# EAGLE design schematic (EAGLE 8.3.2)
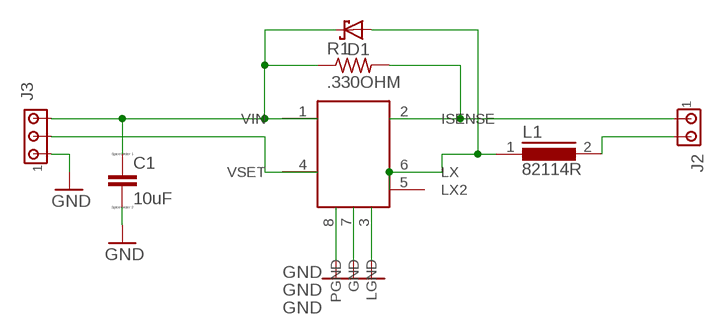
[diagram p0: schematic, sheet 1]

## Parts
C1  10uF  CC1206  [C1206]
D1  SCHOTTKY-DIODESMC  [SMC]
J2  MTA02-156  [1X2MTA]
J3  MTA03-156  [1X3MTA]
L1  82114R  [82114R]
R1  .330OHM  R-US_0207/15  [0207/15]
U$1  PAM2863  [SOP8]

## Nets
GND: C1.2 J3.1 U$1.3(LGND) U$1.7(GND) U$1.8(PGND)
LED+: J2.1 R1.2 U$1.2(ISENSE)
LED-: J2.2 L1.2
N$5: D1.A L1.1 U$1.5(LX2) U$1.6(LX)
VIN: C1.1 D1.C J3.3 R1.1 U$1.1(VIN)
VSET: J3.2 U$1.4(VSET)

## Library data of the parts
C1 = eagle-ltspice:C: CAPACITOR, European symbol; SPICEMODEL: NONE; SPICEPREFIX: C
D1 = diode:SCHOTTKY-DIODE: Schottky Diode
J2 = con-amp:MTA02-156: AMP connector
J3 = con-amp:MTA03-156: AMP connector
L1 = inductors:82114R: INDUCTOR
R1 = rcl:R-US_: RESISTOR, American symbol
U$1 = raccolta:PAM2863: The PAM2863 is a continuous mode inductive step-down converter, designed for driving single or multiple series connected LEDs efficiently from a voltage source higher than the LED voltage. The device operates from an input supply between 4.5V and 40V and provides an externally adjustable output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

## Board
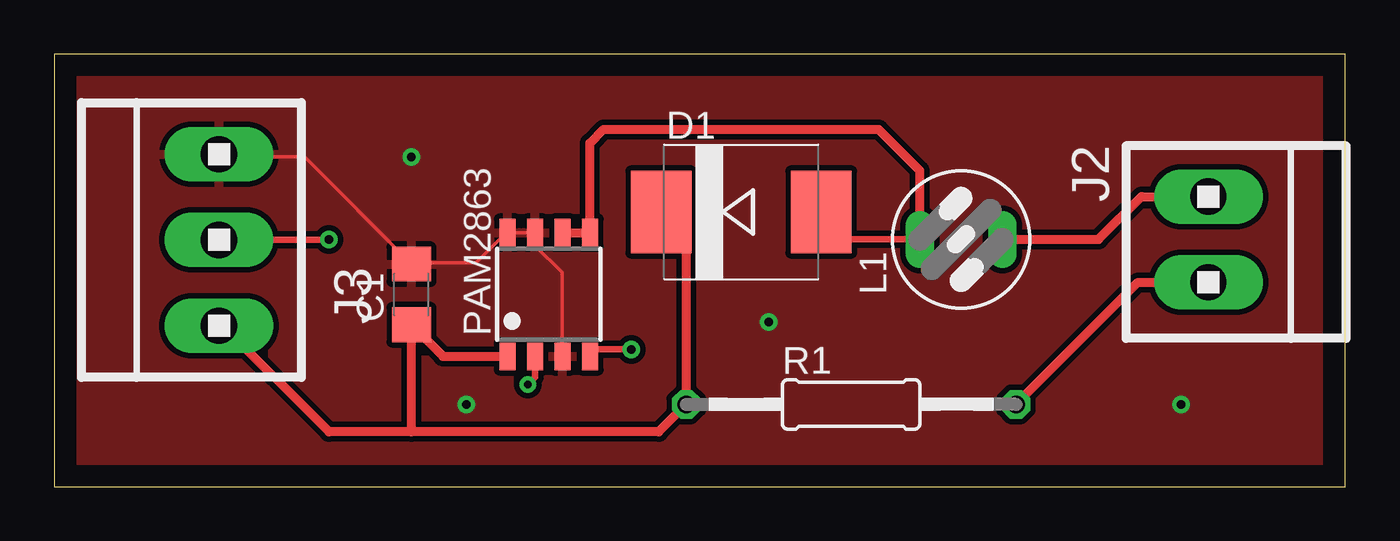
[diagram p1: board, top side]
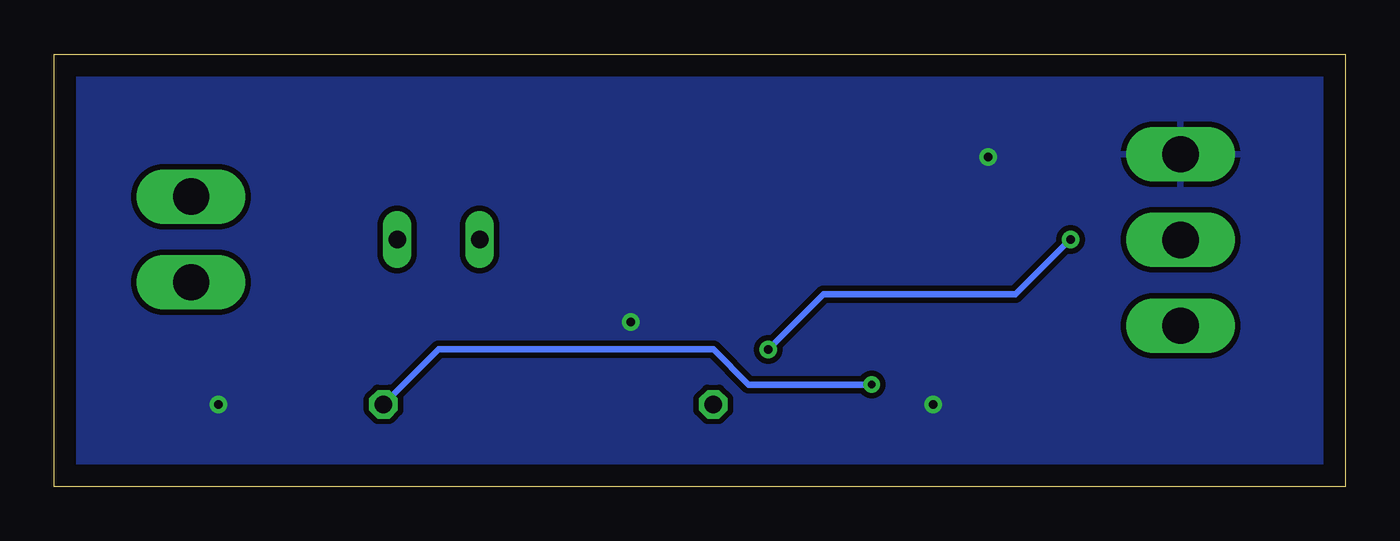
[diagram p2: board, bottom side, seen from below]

Size 59.67 x 19.99 mm. Coordinates in mm from the lower left corner, seen from the top.
Outline: 0,0 59.67,0 59.67,19.99 0,19.99 0,0
Copper layers (1*16): Top 0.035mm / dielectric 1.5mm / Bottom 0.035mm
Design rules "default": minimum track width 6mil, minimum drill 0.35mm, track to track 6mil, track to pad 6mil, pad to pad 6mil, via to via 6mil, smd to smd 6mil, copper to edge 40mil, drill to drill 6mil, minimum pad ring 10mil, minimum via ring 8mil, stop-mask expansion 4mil, vias tented up to drill 0mil, thermal gap 10mil

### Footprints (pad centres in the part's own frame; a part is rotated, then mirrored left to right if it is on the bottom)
C1206 = smd 1.6 x 1.8: 1 -1.4,0; 2 1.4,0
SMC = smd 2.8 x 3.8: A 3.7,0; C -3.7,0
1X2MTA = drill 1.676 long: 1 1.981,0; 2 -1.981,0
1X3MTA = drill 1.676 long: 1 3.937,0; 2 -0.025,0; 3 -3.988,0
82114R = drill 0.813 long: 1 0,1.905; 2 0,-1.905
0207/15 = drill 0.813 octagon: 1 -7.62,0; 2 7.62,0
SOP8 = smd 0.76 x 1.27: 1 -1.905,-2.86; 2 -0.635,-2.86; 3 0.635,-2.86; 4 1.905,-2.86; 5 1.905,2.86; 6 0.635,2.86; 7 -0.635,2.86; 8 -1.905,2.86

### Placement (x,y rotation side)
C1  16.51,8.89 90 top
D1  31.75,12.7 0 top
J2  53.34,11.43 270 top
J3  7.62,11.43 90 top
L1  41.91,11.43 90 top
R1  36.83,3.81 0 top
U$1  22.86,8.89 0 top

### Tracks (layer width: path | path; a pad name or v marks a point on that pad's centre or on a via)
GND  (via drill 0.4)
  Top 0.152: U$1.3 23.47,6.1 23.47,9.91 22.25,11.12 22.25,11.73 U$1.7 22.1,11.73 21.03,11.73 U$1.8 20.88,11.73 19.51,10.36 16.61,10.36 C1.2 16.46,10.36 11.58,15.24 7.62,15.24 J3.1
  other vias: 16.51,15.24 33.02,7.62 19.05,3.81 52.07,3.81
  pour Top (isolate 0.254): 0,20.32 59.69,20.32 59.69,0 0,0
  pour Bottom (isolate 0.254): 0,0 0,20.32 59.69,20.32 59.69,0
LED+  (via drill 0.35)
  Top 0.305: v21.89,4.72 22.23,5.05 U$1.2
  Top 0.406: R1.2 50.09,9.45 J2.1
  Bottom 0.305: v21.89,4.72 27.58,4.72 29.21,6.35 41.91,6.35 R1.2
LED-
  Top 0.406: L1.2 48.26,11.43 50.24,13.41 J2.2
N$5
  Top 0.152: U$1.6 23.62,11.73 | 24.69,11.73 U$1.5
  Top 0.305: D1.A 36.72,11.43 L1.1
  Top 0.406: U$1.5 24.77,15.88 25.4,16.51 38.1,16.51 40.01,14.61 L1.1 | 23.62,11.73 24.69,11.73
VIN
  Top 0.406: D1.C 29.21,11.54 R1.1 27.94,2.54 16.51,2.54 | 16.51,2.54 12.7,2.54 7.8,7.44 J3.3 | 16.51,2.54 C1.1 17.97,6.03 U$1.1
VSET  (via drill 0.4)
  Top 0.305: J3.2 12.68,11.4 v12.7,11.43 | v26.67,6.35 25.09,6.35 U$1.4
  Bottom 0.305: v12.7,11.43 15.24,8.89 24.13,8.89 v26.67,6.35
